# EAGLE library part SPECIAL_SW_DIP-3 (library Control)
DIP SWITCH
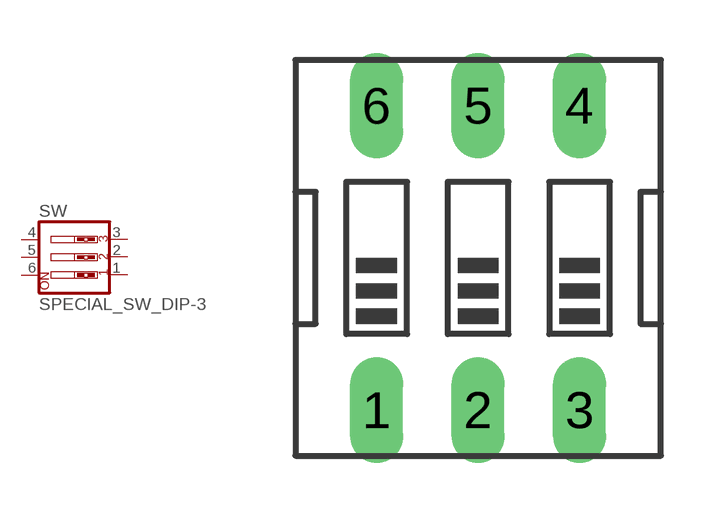
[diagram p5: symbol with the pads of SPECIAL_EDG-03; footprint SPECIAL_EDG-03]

Designator prefix SW

## SPECIAL_SW_DIP-3  [SPECIAL_EDG-03]
1  1  pas
2  2  pas
3  3  pas
4  4  pas
5  5  pas
6  6  pas

## Footprint SPECIAL_EDG-03 (pad centres in mm)
DIP SWITCH
drill 0.813 long: 1 -2.54,-3.81; 2 0,-3.81; 3 2.54,-3.81; 4 2.54,3.81; 5 0,3.81; 6 -2.54,3.81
